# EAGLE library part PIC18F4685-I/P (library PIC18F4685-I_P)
Check availability
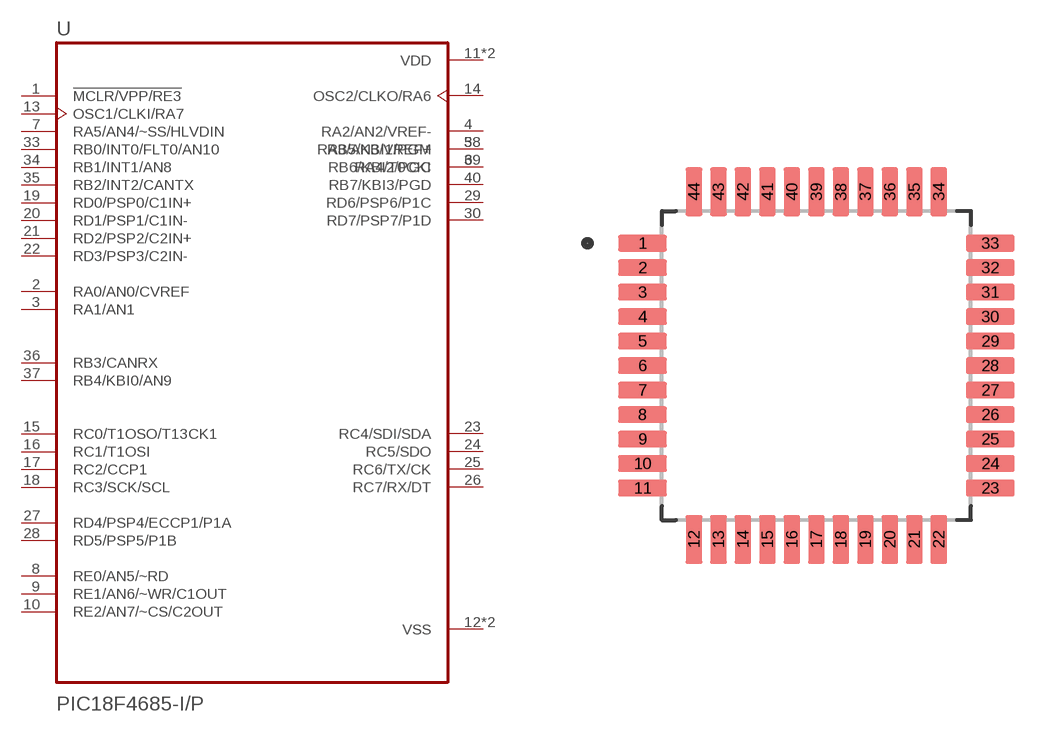
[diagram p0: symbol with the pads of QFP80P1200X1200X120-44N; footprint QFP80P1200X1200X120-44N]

Designator prefix -

## PIC18F4685-I/P (Availability: In Stock; Description: PIC PIC® 18F Microcontroller IC 8-Bit 40MHz 96KB (48K x 16) FLASH 44-TQFP (10x10); MF: Microchip; MP: PIC18F4685-I/P; Package: DIP-40 Microchip Technology; Price: None; Purchase-URL: https://pricing.snapeda.com/search/part/PIC18F4685-I/P/?ref=eda)  [QFP80P1200X1200X120-44N]
1  !MCLR/VPP/RE3  in
2  RA0/AN0/CVREF
3  RA1/AN1
4  RA2/AN2/VREF-
5  RA3/AN3/VREF+
6  RA4/T0CKI
7  RA5/AN4/~SS/HLVDIN  in
8  RE0/AN5/~RD
9  RE1/AN6/~WR/C1OUT
10  RE2/AN7/~CS/C2OUT
11  VDD  pwr
12  VSS  pwr
13  OSC1/CLKI/RA7  in
14  OSC2/CLKO/RA6  out
15  RC0/T1OSO/T13CK1
16  RC1/T1OSI
17  RC2/CCP1
18  RC3/SCK/SCL
19  RD0/PSP0/C1IN+  in
20  RD1/PSP1/C1IN-  in
21  RD2/PSP2/C2IN+  in
22  RD3/PSP3/C2IN-  in
23  RC4/SDI/SDA
24  RC5/SDO
25  RC6/TX/CK
26  RC7/RX/DT
27  RD4/PSP4/ECCP1/P1A
28  RD5/PSP5/P1B
29  RD6/PSP6/P1C
30  RD7/PSP7/P1D
31  VSS  pwr
32  VDD  pwr
33  RB0/INT0/FLT0/AN10  in
34  RB1/INT1/AN8  in
35  RB2/INT2/CANTX  in
36  RB3/CANRX
37  RB4/KBI0/AN9
38  RB5/KBI1/PGM
39  RB6/KBI2/PGC
40  RB7/KBI3/PGD

## Footprint QFP80P1200X1200X120-44N (pad centres in mm)
smd 1.6 x 0.55: 1 -5.68,4; 2 -5.68,3.2; 3 -5.68,2.4; 4 -5.68,1.6; 5 -5.68,0.8; 6 -5.68,0; 7 -5.68,-0.8; 8 -5.68,-1.6; 9 -5.68,-2.4; 10 -5.68,-3.2; 11 -5.68,-4; 23 5.68,-4; 24 5.68,-3.2; 25 5.68,-2.4; 26 5.68,-1.6; 27 5.68,-0.8; 28 5.68,0; 29 5.68,0.8; 30 5.68,1.6; 31 5.68,2.4; 32 5.68,3.2; 33 5.68,4
smd 0.55 x 1.6: 12 -4,-5.68; 13 -3.2,-5.68; 14 -2.4,-5.68; 15 -1.6,-5.68; 16 -0.8,-5.68; 17 0,-5.68; 18 0.8,-5.68; 19 1.6,-5.68; 20 2.4,-5.68; 21 3.2,-5.68; 22 4,-5.68; 34 4,5.68; 35 3.2,5.68; 36 2.4,5.68; 37 1.6,5.68; 38 0.8,5.68; 39 0,5.68; 40 -0.8,5.68; 41 -1.6,5.68; 42 -2.4,5.68; 43 -3.2,5.68; 44 -4,5.68

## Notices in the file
This work is licensed under a Creative Commons Attribution-ShareAlike 4.0 International License (CC BY-SA) with Design Exception 1.0
